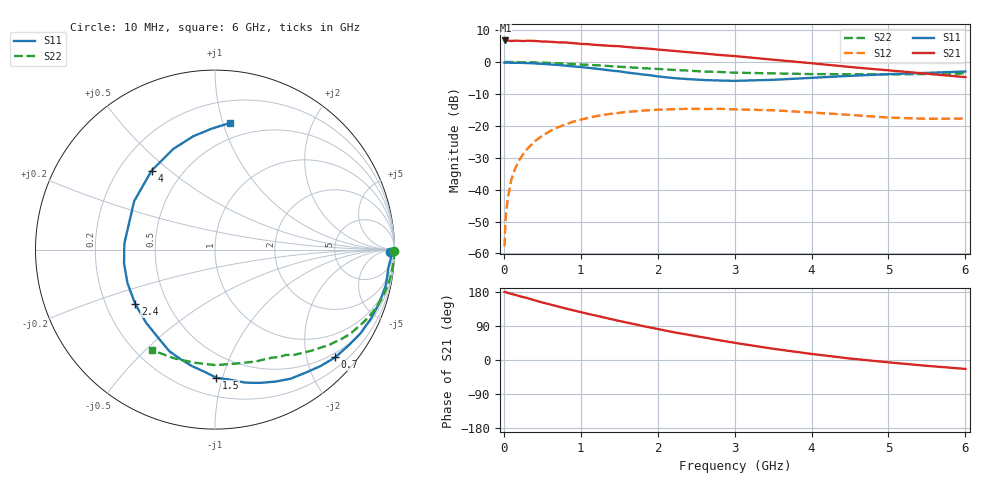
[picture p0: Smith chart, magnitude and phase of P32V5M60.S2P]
! SIEMENS Small Signal Semiconductors
! BFP181
! Si NPN RF Bipolar Junction Transistor in SOT143
! VCE = 2.5 V  IC = 0.6 mA
! Common Emitter S-Parameters:  March  1996
# GHz  S  MA  R  50
!  f  S11  S21  S12  S22
! GHz  MAG  ANG  MAG  ANG  MAG  ANG  MAG  ANG
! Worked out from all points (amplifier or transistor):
!   36 points, 10 MHz to 6 GHz, reference 50 ohm
!   highest |S21| = 6.7 dB at 20 MHz (marker M1)
!   |S21| within 3 dB of that: start of sweep to 2.076 GHz
!   unconditionally stable (mu >= 1): 3.619 GHz to end of sweep
!   at 250 MHz: K = 0.08, MSG = 17.7 dB, |S12| = -28.9 dB
!   at 1.4 GHz: K = 0.44, MSG = 10.6 dB, |S12| = -16.2 dB
!   at 6 GHz: K = 1.43, MAG = 2.6 dB, |S12| = -17.7 dB
!   S11 on the Smith chart (normalised r, x): 10 MHz: 61, -34; 700 MHz: 0.41, -2.56; 1.5 GHz: 0.33, -0.95; 2.4 GHz: 0.33, -0.28; 4 GHz: 0.34, +0.43; 6 GHz: 0.37, +1.05
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0.01  0.9751 -0.8  2.151 179.8  0.0013 88.9  1 -0.3
0.02  0.9796 -1.1  2.174 179.5  0.0032 85.0  0.999 -0.6
0.05  0.9805 -3.0  2.173 177.2  0.0072 89.7  0.9979 -1.5
0.1  0.9713 -5.9  2.131 174.5  0.0147 85.0  0.9983 -2.9
0.15  0.9713 -9.2  2.159 171.6  0.0218 82.9  0.9952 -4.3
0.2  0.9717 -12.1  2.151 168.8  0.029 81.8  0.9942 -5.8
0.3  0.9621 -18.2  2.151 163.8  0.0428 77.1  0.9898 -8.6
0.4  0.9497 -24.0  2.138 157.5  0.057 73.2  0.984 -11.5
0.7  0.899 -41.9  2.031 141.4  0.0943 60.9  0.9544 -19.6
0.8  0.8757 -47.8  2.022 136.2  0.1051 57.1  0.943 -22.2
1.1  0.8093 -65.3  1.9 121.4  0.1336 46.1  0.9009 -29.3
1.5  0.7134 -89.5  1.767 103.1  0.1596 33.3  0.8419 -37.8
1.8  0.6389 -107.8  1.644 89.8  0.1728 25.3  0.8014 -43.1
2.2  0.5602 -133.1  1.495 73.6  0.1817 15.2  0.7522 -50.0
2.4  0.5385 -145.6  1.422 66.5  0.1846 10.7  0.733 -53.2
2.6  0.5221 -159.1  1.358 59.5  0.1834 7.3  0.7077 -56.0
3  0.5062 176.2  1.238 45.3  0.181 -0.4  0.6799 -62.3
3.5  0.525 149.1  1.086 29.7  0.1751 -7.3  0.6632 -70.1
4  0.5643 128.8  0.956 16.0  0.1617 -12.4  0.646 -79.4
4.5  0.6067 112.7  0.835 3.9  0.1483 -15.9  0.6438 -89.6
5.5  0.675 91.3  0.656 -15.4  0.1289 -11.7  0.6476 -111.1
6  0.7097 83.4  0.579 -23.5  0.1298 -8.3  0.6607 -122.2
